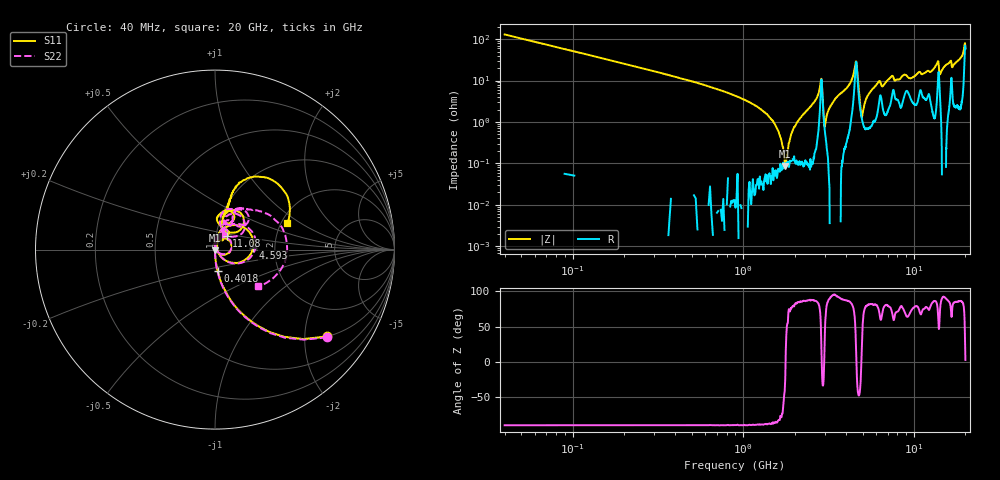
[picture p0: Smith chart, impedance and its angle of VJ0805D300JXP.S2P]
! VJ0805D300JXP
! DATE 10/29/2021  12:26
! CAPACITORS MOUNTED IN SERIES ON 25 MIL THICK MICROSTRIP SUBSTRATE
# GHz  S  MA  R  50.00
!  FREQ  S11M  S11A  S21M  S21A  S12M  S12A  S22M  S22A
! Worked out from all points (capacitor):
!   1601 points, 40 MHz to 20 GHz, reference 50 ohm
!   read as one part in series: C = 30.7 pF near 139.8 MHz
!   lowest |Z| = 86.8 mohm at 1.762 GHz (marker M1)
!   series resonance near 1.768 GHz, so ESL is about 260 pH
!   S11 on the Smith chart (normalised r, x): 40 MHz: 1.00, -2.58; 401.8 MHz: 1.00, -0.24; 4.593 GHz: 1.54, +0.03; 11.08 GHz: 1.12, +0.18; 20 GHz: 2.15, +0.77
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0.04  0.7896 -37.8  0.6107 52.1  0.6099 52.2  0.793 -38.1
0.401775  0.1211 -83.0  0.9919 6.9  0.9931 6.9  0.1231 -83.5
1.4372  0.01494 -88.3  0.9993 0.6  0.9992 0.5  0.01539 -88.4
1.76155  0.003307 -77.8  0.9988 -0.1  0.9996 -0.2  0.003362 -73.9
1.898775  0.001644 35.7  0.9987 -0.4  0.999 -0.5  0.001665 59.1
2.1358  0.00857 87.7  0.9984 -0.9  0.9986 -0.9  0.007936 79.0
2.80945  0.06098 67.5  0.9794 -3.9  0.9804 -3.9  0.06219 71.1
3.05895  0.007467 60.2  0.9961 -0.9  0.9968 -1.0  0.008025 69.5
3.370825  0.02109 91.6  1.002 -2.1  1.003 -2.2  0.02709 97.4
4.593375  0.213 2.3  0.7803 -1.4  0.7813 -1.5  0.2259 1.7
4.992575  0.01262 20.3  0.9892 -0.9  0.9901 -1.1  0.009809 30.8
5.70365  0.04923 68.0  0.9886 -3.8  0.9908 -4.0  0.06091 84.5
6.70165  0.07249 73.1  0.982 -4.9  0.9827 -5.0  0.07258 71.5
10.02  0.1067 68.3  0.9675 -7.4  0.9687 -7.6  0.1131 69.5
11.08038  0.1012 50.1  0.9463 -7.8  0.9472 -8.1  0.1486 67.4
13.35083  0.1967 74.4  0.9656 -13.2  0.9658 -13.4  0.1914 72.0
13.8124  0.2489 57.7  0.881 -15.1  0.8818 -15.5  0.2336 49.3
14.14922  0.1205 54.7  0.9385 -8.0  0.9393 -8.2  0.1061 57.7
15.19712  0.1749 86.6  0.9814 -14.1  0.9819 -14.3  0.2363 71.9
16.68165  0.1629 64.1  0.9156 -12.2  0.9165 -12.5  0.1807 47.0
19.4511  0.4131 68.1  0.8509 -27.5  0.8524 -27.8  0.327 41.0
20  0.4279 20.1  0.594 -4.6  0.5937 -4.8  0.3134 -40.9
